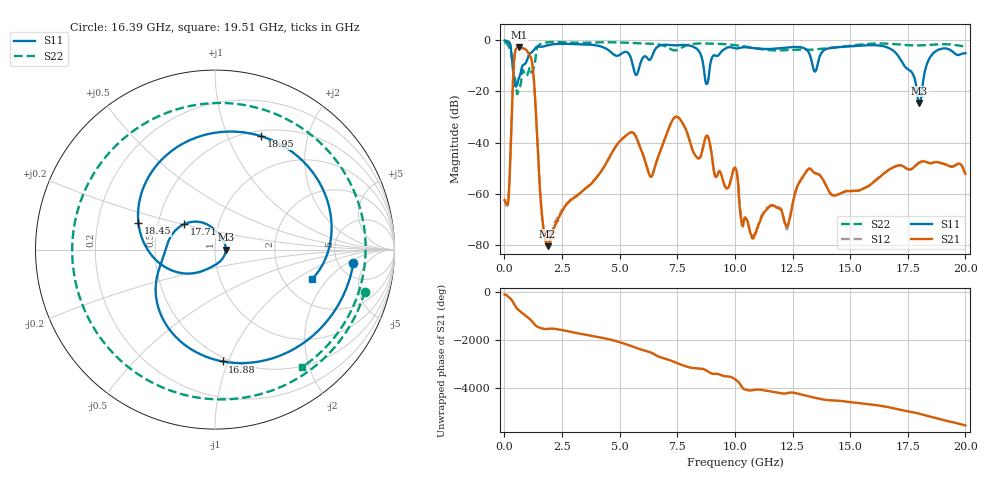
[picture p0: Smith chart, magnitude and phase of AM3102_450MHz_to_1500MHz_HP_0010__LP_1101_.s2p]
!Agilent Technologies,E8364B,MY43040894,A.07.50.67
!Agilent E8364B: A.07.50.67
!Date: Thursday, January 11, 2018 05:28:54
!Correction: S11(Full 2 Port(1,2))
!S21(Full 2 Port(1,2))
!S12(Full 2 Port(1,2))
!S22(Full 2 Port(1,2))
!S2P File: Measurements: S11, S21, S12, S22:
# Hz S  dB  R 50
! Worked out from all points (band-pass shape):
!   1601 points, 10 MHz to 20 GHz, reference 50 ohm
!   highest |S21| = -2.77 dB at 634.7 MHz (marker M1); lowest = -80.5 dB at 1.872 GHz (marker M2)
!   |S21| within 3 dB of the highest: 445 MHz to 1.094 GHz (649.2 MHz wide, 84.4 % of centre)
!   lowest |S11| = -24.5 dB at 18 GHz (marker M3), VSWR 1.13, Z = 56.4 + j0.00893 ohm
!   |S11| at or under -10 dB: 357.1 MHz to 781.5 MHz (424.4 MHz wide, 74.5 % of centre); 5.577 GHz to 5.87 GHz (292.2 MHz wide, 5.11 % of centre); 17.35 GHz to 18.31 GHz (951.2 MHz wide, 5.34 % of centre)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
!   |S22| runs from -21.0 to -0.6 dB; largest |S21 - S12| = 0.0019
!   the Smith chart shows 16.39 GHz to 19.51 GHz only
!   S11 on the Smith chart (normalised r, x): 16.39 GHz: 6.93, -2.55; 16.88 GHz: 0.47, -0.95; 17.71 GHz: 0.68, +0.20; 18.45 GHz: 0.39, +0.14; 18.95 GHz: 0.56, +1.33; 19.51 GHz: 2.87, -1.38
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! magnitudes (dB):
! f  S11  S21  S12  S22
! 10 MHz  -0.1  -62.4  -63.7  -0.6
! 634.7 MHz  -14.7  -2.8  -2.8  -19.1
! 1.197 GHz  -4.6  -8.4  -8.4  -12.5
! 1.609 GHz  -2.5  -66.2  -66.4  -1.3
! 1.872 GHz  -2.0  -80.5  -79.9  -0.8
! 3.346 GHz  -1.5  -59.2  -59.2  -1.0
! 5.432 GHz  -5.7  -36.2  -36.2  -1.0
! 6.682 GHz  -2.3  -45.3  -45.3  -1.6
! 7.481 GHz  -2.0  -29.9  -29.9  -3.8
! 8.781 GHz  -17.1  -37.3  -37.3  -1.3
! 10.01 GHz  -3.1  -49.8  -49.8  -1.9
! 10.79 GHz  -3.0  -77.5  -77.0  -3.0
! 13.34 GHz  -8.6  -50.8  -50.8  -3.7
! 16.39 GHz  -2.2  -52.7  -52.6  -1.2
! 16.68 GHz  -3.0  -50.7  -50.6  -1.3
! 16.88 GHz  -4.1  -49.6  -49.6  -1.5
! 17.71 GHz  -13.0  -50.0  -50.0  -2.0
! 18 GHz  -24.5  -47.8  -47.8  -2.0
! 18.45 GHz  -6.9  -48.0  -48.0  -1.8
! 18.95 GHz  -3.3  -48.0  -48.0  -1.5
! 19.51 GHz  -5.0  -49.2  -49.1  -1.8
! 20 GHz  -5.1  -52.2  -52.2  -2.4
